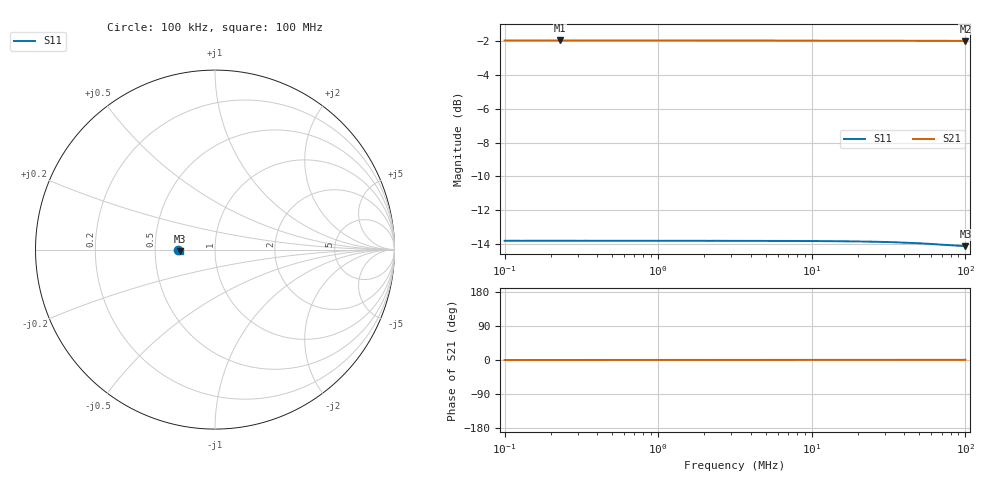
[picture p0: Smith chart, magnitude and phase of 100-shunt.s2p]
! ListType=Log
!!100 Ohm Shunt
# MHZ S RI R 50
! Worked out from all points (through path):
!   200 points, 100 kHz to 100 MHz, reference 50 ohm
!   highest |S21| = -1.95 dB at 230 kHz (marker M1); lowest = -2.0 dB at 100 MHz (marker M2)
!   lowest |S11| = -14.1 dB at 100 MHz (marker M3), VSWR 1.49, Z = 33.6 - j0.647 ohm
!   |S11| at or under -10 dB: start of sweep to end of sweep
!   S12 and S22 are empty: the file has one direction only
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0.1  -0.2038 3.77e-05  0.7986 -4.7e-06  0 0  0 0
0.230043  -0.2038 2.3e-05  0.7987 -1.29e-05  0 0  0 0
0.3255089  -0.2038 -2.5e-06  0.7986 -1.7e-06  0 0  0 0
0.3370064  -0.2039 2.37e-05  0.7986 4.4e-06  0 0  0 0
0.3489101  -0.2038 9.7e-06  0.7986 -4.7e-06  0 0  0 0
1.023411  -0.2038 0.000114  0.7986 1.75e-05  0 0  0 0
2.121452  -0.2037 0.000131  0.7986 6.18e-05  0 0  0 0
2.354286  -0.2038 6.61e-05  0.7986 6.86e-05  0 0  0 0
2.70496  -0.2037 0.000105  0.7986 9.69e-05  0 0  0 0
3.107866  -0.2038 8.51e-05  0.7986 9.91e-05  0 0  0 0
3.217642  -0.2037 0.000169  0.7986 8.03e-05  0 0  0 0
4.397604  -0.2038 0.000159  0.7986 0.000151  0 0  0 0
5.231099  -0.2036 0.000129  0.7985 0.00018  0 0  0 0
6.010277  -0.2037 0.000131  0.7985 0.000193  0 0  0 0
10.11638  -0.2035 0.000134  0.7985 0.000373  0 0  0 0
20.25502  -0.2029 -9.2e-05  0.7983 0.000873  0 0  0 0
31.80626  -0.202 -0.000565  0.7981 0.00153  0 0  0 0
45.00558  -0.2009 -0.00134  0.7977 0.00234  0 0  0 0
59.41134  -0.1995 -0.00271  0.7973 0.00338  0 0  0 0
81.19845  -0.1975 -0.00577  0.7966 0.00523  0 0  0 0
93.29304  -0.1966 -0.00789  0.7963 0.00635  0 0  0 0
100  -0.1962 -0.00926  0.7962 0.00704  0 0  0 0
